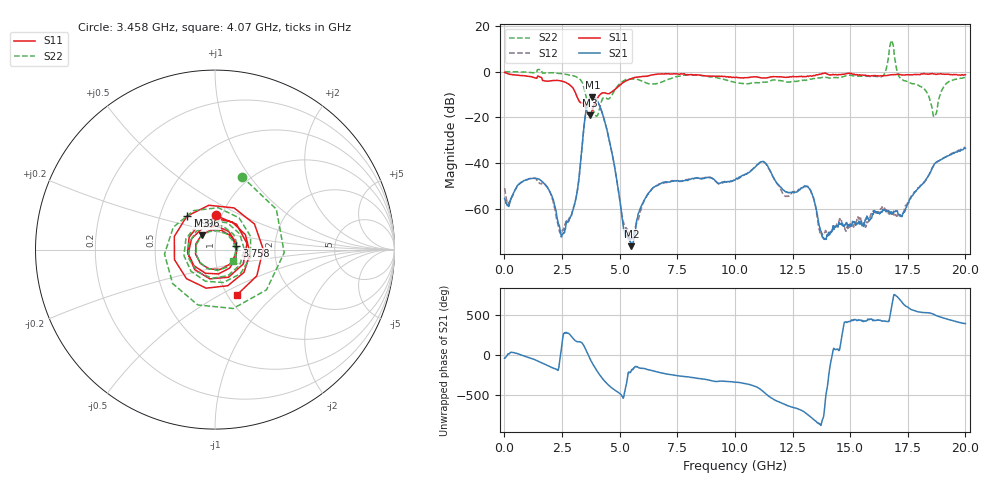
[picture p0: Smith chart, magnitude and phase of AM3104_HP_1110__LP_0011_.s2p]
!Created with skrf (http://scikit-rf.org).
# Hz S RI R 50.0
!freq ReS11 ImS11 ReS21 ImS21 ReS12 ImS12 ReS22 ImS22
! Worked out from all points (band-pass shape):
!   1601 points, 10 MHz to 20 GHz, reference 50 ohm
!   highest |S21| = -11.14 dB at 3.821 GHz (marker M1); lowest = -76.2 dB at 5.507 GHz (marker M2)
!   |S21| within 3 dB of the highest: 3.604 GHz to 4.099 GHz (495.6 MHz wide, 12.9 % of centre)
!   lowest |S11| = -19.1 dB at 3.708 GHz (marker M3), VSWR 1.25, Z = 42.5 + j7.09 ohm
!   |S11| at or under -10 dB: 3.112 GHz to 4.161 GHz (1.049 GHz wide, 28.9 % of centre)
!   |S22| runs from -19.8 to 13.6 dB; largest |S21 - S12| = 0.013
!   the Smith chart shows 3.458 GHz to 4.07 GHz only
!   S11 on the Smith chart (normalised r, x): 3.458 GHz: 0.94, +0.37; 3.758 GHz: 1.27, +0.05; 3.996 GHz: 0.69, +0.27; 4.07 GHz: 1.10, -0.61
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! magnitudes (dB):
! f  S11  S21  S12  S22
! 10 MHz  -0.4  -55.4  -50.9  0.0
! 1.534 GHz  -2.3  -47.1  -48.8  0.9
! 2.546 GHz  -4.3  -70.8  -69.0  -1.0
! 3.071 GHz  -9.0  -56.9  -56.8  -2.1
! 3.346 GHz  -13.6  -35.3  -35.5  -4.2
! 3.458 GHz  -14.4  -23.5  -23.5  -7.3
! 3.708 GHz  -19.1  -11.7  -11.8  -15.4
! 3.758 GHz  -18.3  -11.3  -11.4  -15.8
! 3.821 GHz  -16.6  -11.1  -11.2  -16.2
! 3.996 GHz  -12.3  -12.4  -12.4  -19.5
! 4.07 GHz  -11.0  -13.6  -13.6  -18.4
! 5.507 GHz  -3.1  -76.2  -72.8  -3.3
! 6.682 GHz  -1.1  -49.6  -49.3  -5.1
! 10.01 GHz  -2.7  -47.4  -47.3  -4.7
! 11.2 GHz  -2.8  -39.3  -39.4  -4.7
! 12.17 GHz  -2.5  -52.2  -54.3  -4.3
! 13.34 GHz  -2.0  -53.3  -53.5  -3.3
! 13.88 GHz  -0.7  -72.8  -70.6  -2.5
! 16.35 GHz  -1.8  -61.2  -59.9  -2.3
! 16.68 GHz  -1.5  -61.1  -62.1  7.1
! 18.66 GHz  -1.0  -40.2  -40.2  -19.5
! 20 GHz  -1.4  -33.5  -33.0  -2.6
